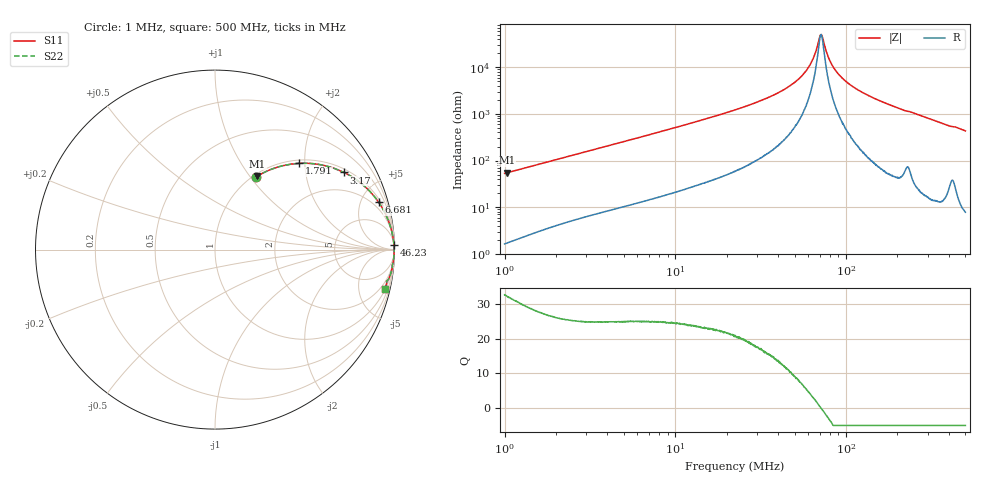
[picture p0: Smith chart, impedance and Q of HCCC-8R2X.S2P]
!s-Parameter Generated by FASTRON Sdn. Bhd.
!FASTRON P/N : HCCC-8R2X
!Keysight Technologies,E4991B,MY54100416,A.01.15
!Date: Thu Apr 02 16:05:47 2026
!Version  : Rev00 Thu Apr 02 16:05:47 2026
!Data & Calibration Information:
!PortZ  Port1:50+j0  Port2:50+j0
!When reading, reference impedance value at option line is always used.
! Remarks : This data is being provided solely for informational purposes.
!Freq	S11	S21	S12	S22
# Hz S dB R 50
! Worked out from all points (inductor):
!   1601 points, 1 MHz to 500 MHz, reference 50 ohm
!   read as one part in series: L = 8.38 uH near 1.032 MHz
!   highest Q = 32.2 at 1.032 MHz (marker M1), where L = 8.42 uH
!   self-resonance near 71.15 MHz
!   S11 on the Smith chart (normalised r, x): 1 MHz: 1.03, +1.06; 1.791 MHz: 1.07, +1.87; 3.17 MHz: 1.13, +3.26; 6.681 MHz: 1.27, +6.79; 46.23 MHz: 8, +77; 500 MHz: 1.16, -8.67
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1000000  -6.70 60.7  -1.18 -27.5  -1.18 -27.5  -6.70 60.7
1031561  -6.50 60.0  -1.25 -28.2  -1.25 -28.2  -6.50 60.0
1790723  -3.46 45.7  -2.90 -42.1  -2.90 -42.1  -3.46 45.7
2820919  -1.84 33.7  -5.11 -54.0  -5.11 -54.0  -1.84 33.7
3169541  -1.54 30.8  -5.79 -56.8  -5.79 -56.8  -1.54 30.8
6681481  -0.45 16.2  -11.08 -71.5  -11.08 -71.5  -0.45 16.2
7957584  -0.34 13.7  -12.48 -73.9  -12.48 -73.9  -0.34 13.7
2.236068e7  -0.06 4.7  -21.79 -82.6  -21.79 -82.6  -0.06 4.7
3.441328e7  -0.03 2.6  -26.84 -83.7  -26.84 -83.7  -0.03 2.6
4.623034e7  -0.02 1.5  -31.77 -83.2  -31.77 -83.2  -0.02 1.5
5.570526e7  -0.02 0.8  -36.75 -80.6  -36.75 -80.6  -0.02 0.8
6.307767e7  -0.02 0.4  -42.60 -73.5  -42.60 -73.5  -0.02 0.4
6.608728e7  -0.02 0.3  -46.20 -65.3  -46.20 -65.3  -0.02 0.3
6.978047e7  -0.02 0.1  -52.49 -33.3  -52.49 -33.3  -0.02 0.1
7.170375e7  -0.02 -0.0  -53.97 8.1  -53.97 8.1  -0.02 -0.0
7.310989e7  -0.02 -0.1  -52.47 34.0  -52.47 34.0  -0.02 -0.1
7.749595e7  -0.02 -0.3  -45.74 67.6  -45.74 67.6  -0.02 -0.3
8.150948e7  -0.02 -0.4  -41.95 75.1  -41.95 75.1  -0.02 -0.4
9.447321e7  -0.02 -1.0  -35.55 82.4  -35.55 82.4  -0.02 -1.0
1.206648e8  -0.02 -1.8  -29.84 85.0  -29.84 85.0  -0.02 -1.8
1.77937e8  -0.03 -3.6  -24.10 84.6  -24.10 84.6  -0.03 -3.6
5e8  -0.26 -12.9  -13.00 76.0  -13.00 76.0  -0.26 -12.9
